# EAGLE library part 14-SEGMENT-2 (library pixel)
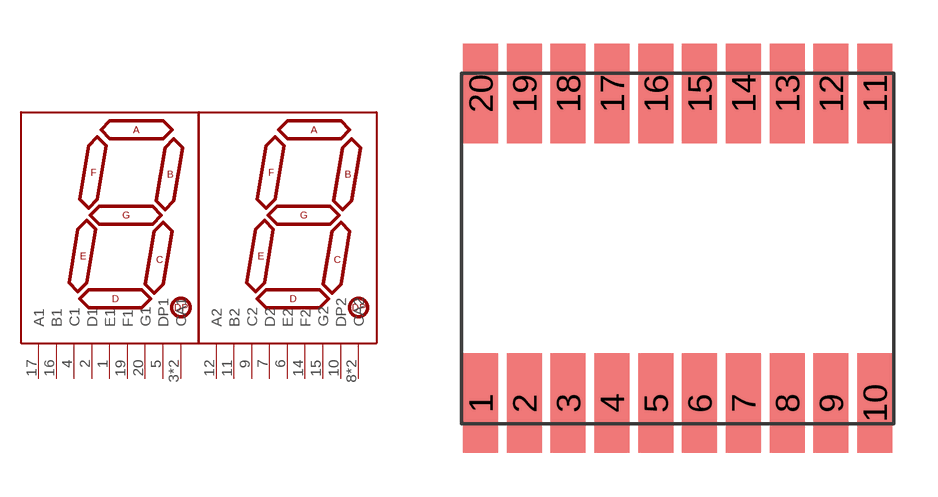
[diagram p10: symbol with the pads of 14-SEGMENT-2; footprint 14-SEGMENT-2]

Designator prefix -

## 14-SEGMENT-2  [14-SEGMENT-2]
1  E1
2  D1
3  CA1
4  C1
5  DP1
6  E2
7  D2
8  CA2
9  C2
10  DP2
11  B2
12  A2
13  CA2
14  F2
15  G2
16  B1
17  A1
18  CA1
19  F1
20  G1

## Footprint 14-SEGMENT-2 (pad centres in mm)
smd 1.2 x 3.4: 1 -6.75,-5.3; 2 -5.25,-5.3; 3 -3.75,-5.3; 4 -2.25,-5.3; 5 -0.75,-5.3; 6 0.75,-5.3; 7 2.25,-5.3; 8 3.75,-5.3; 9 5.25,-5.3; 10 6.75,-5.3; 11 6.75,5.3; 12 5.25,5.3; 13 3.75,5.3; 14 2.25,5.3; 15 0.75,5.3; 16 -0.75,5.3; 17 -2.25,5.3; 18 -3.75,5.3; 19 -5.25,5.3; 20 -6.75,5.3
